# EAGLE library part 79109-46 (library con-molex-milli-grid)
RECEPTACAL
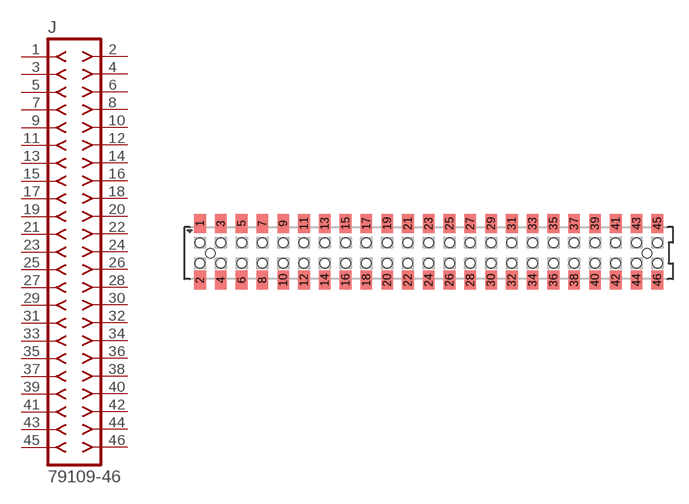
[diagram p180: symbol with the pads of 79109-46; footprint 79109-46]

Designator prefix J

## 79109-46  [79109-46]
1  1  pas
2  2  pas
3  3  pas
4  4  pas
5  5  pas
6  6  pas
7  7  pas
8  8  pas
9  9  pas
10  10  pas
11  11  pas
12  12  pas
13  13  pas
14  14  pas
15  15  pas
16  16  pas
17  17  pas
18  18  pas
19  19  pas
20  20  pas
21  21  pas
22  22  pas
23  23  pas
24  24  pas
25  25  pas
26  26  pas
27  27  pas
28  28  pas
29  29  pas
30  30  pas
31  31  pas
32  32  pas
33  33  pas
34  34  pas
35  35  pas
36  36  pas
37  37  pas
38  38  pas
39  39  pas
40  40  pas
41  41  pas
42  42  pas
43  43  pas
44  44  pas
45  45  pas
46  46  pas

## Footprint 79109-46 (pad centres in mm)
RECEPTACAL SMD Dual Row, Vertical, Pass-Thru
smd 1.12 x 1.83: 1 -22,2.85; 2 -22,-2.6; 3 -20,2.85; 4 -20,-2.6; 5 -18,2.85; 6 -18,-2.6; 7 -16,2.85; 8 -16,-2.6; 9 -14,2.85; 10 -14,-2.6; 11 -12,2.85; 12 -12,-2.6; 13 -10,2.85; 14 -10,-2.6; 15 -8,2.85; 16 -8,-2.6; 17 -6,2.85; 18 -6,-2.6; 19 -4,2.85; 20 -4,-2.6; 21 -2,2.85; 22 -2,-2.6; 23 0,2.85; 24 0,-2.6; 25 2,2.85; 26 2,-2.6; 27 4,2.85; 28 4,-2.6; 29 6,2.85; 30 6,-2.6; 31 8,2.85; 32 8,-2.6; 33 10,2.85; 34 10,-2.6; 35 12,2.85; 36 12,-2.6; 37 14,2.85; 38 14,-2.6; 39 16,2.85; 40 16,-2.6; 41 18,2.85; 42 18,-2.6; 43 20,2.85; 44 20,-2.6; 45 22,2.85; 46 22,-2.6
hole 0.914 at -21,0
hole 0.914 at -22,1
hole 0.914 at -22,-1
hole 0.914 at -20,-1
hole 0.914 at -20,1
hole 0.914 at -18,-1
hole 0.914 at -18,1
hole 0.914 at -16,1
hole 0.914 at -16,-1
hole 0.914 at -14,1
hole 0.914 at -14,-1
hole 0.914 at -12,1
hole 0.914 at -12,-1
hole 0.914 at -10,1
hole 0.914 at -10,-1
hole 0.914 at -8,-1
hole 0.914 at -8,1
hole 0.914 at -6,1
hole 0.914 at -6,-1
hole 0.914 at -4,1
hole 0.914 at -4,-1
hole 0.914 at -2,1
hole 0.914 at -2,-1
hole 0.914 at 0,-1
hole 0.914 at 0,1
hole 0.914 at 2,1
hole 0.914 at 4,1
hole 0.914 at 6,1
hole 0.914 at 2,-1
hole 0.914 at 4,-1
hole 0.914 at 6,-1
hole 0.914 at 8,-1
hole 0.914 at 10,-1
hole 0.914 at 12,-1
hole 0.914 at 14,-1
hole 0.914 at 16,-1
hole 0.914 at 8,1
hole 0.914 at 10,1
hole 0.914 at 12,1
hole 0.914 at 14,1
hole 0.914 at 16,1
hole 0.914 at 18,-1
hole 0.914 at 20,-1
hole 0.914 at 18,1
hole 0.914 at 20,1
hole 0.914 at 22,1
hole 0.914 at 22,-1
hole 0.914 at 21,0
